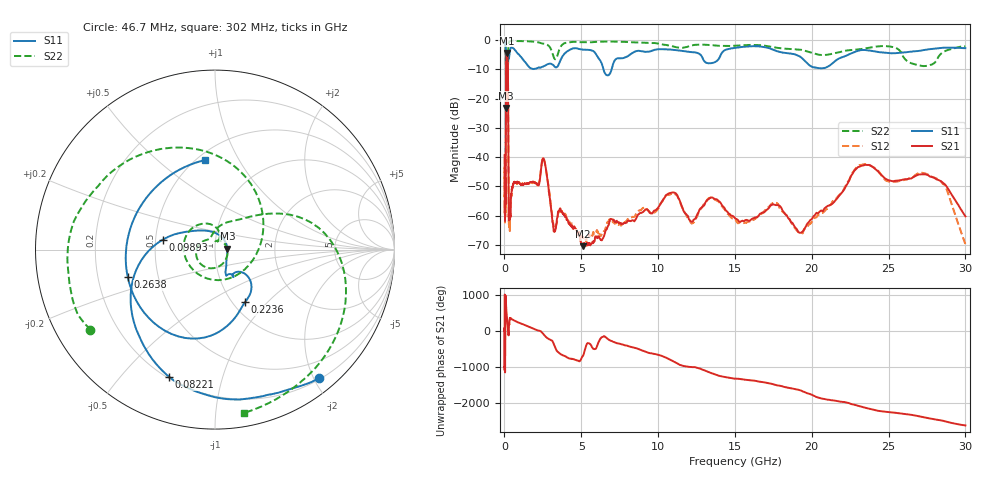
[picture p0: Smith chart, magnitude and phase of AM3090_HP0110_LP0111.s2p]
! Date/Time: Thu, Feb 28, 2019 1:59 PM
! Network Analyzer: Agilent Technologies E8364B Rev: A.07.50.67
! Sweep from 0.010 to 30.000 GHz, 1601 Points, Sweep Type: LOG
! Power Supply: 5.023 V, 0.002 A
# Hz S DB R 50
!freq MagS11 AngS11 MagS21 AngS21 MagS12 AngS12 MagS22 AngS22
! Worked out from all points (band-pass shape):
!   1601 points, 10 MHz to 30 GHz, reference 50 ohm
!   highest |S21| = -4.45 dB at 156 MHz (marker M1); lowest = -70.4 dB at 5.103 GHz (marker M2)
!   |S21| within 3 dB of the highest: 110.9 MHz to 217.7 MHz (106.8 MHz wide, 65 % of centre)
!   lowest |S11| = -23.2 dB at 107.7 MHz (marker M3), VSWR 1.15, Z = 57.4 + j0.698 ohm
!   |S11| at or under -10 dB: 98.52 MHz to 217.9 MHz (119.4 MHz wide, 75.5 % of centre); 6.446 GHz to 6.977 GHz (531.2 MHz wide, 7.91 % of centre)
!   |S22| runs from -28.5 to -0.2 dB; largest |S21 - S12| = 0.015
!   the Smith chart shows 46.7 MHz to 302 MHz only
!   S11 on the Smith chart (normalised r, x): 46.7 MHz: 0.22, -2.08; 82.21 MHz: 0.21, -0.68; 98.93 MHz: 0.55, +0.07; 223.6 MHz: 1.14, -0.75; 263.8 MHz: 0.33, -0.14; 302 MHz: 0.55, +0.73
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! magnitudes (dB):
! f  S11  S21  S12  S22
! 10 MHz  -0.2  -39.3  -49.0  -0.5
! 38.04 MHz  -0.5  -59.8  -61.8  -1.4
! 46.7 MHz  -0.7  -48.1  -51.7  -1.7
! 82.21 MHz  -2.5  -52.0  -53.7  -4.9
! 98.93 MHz  -10.6  -17.5  -17.5  -15.5
! 107.7 MHz  -23.2  -8.7  -8.7  -15.1
! 144.7 MHz  -16.1  -4.6  -4.5  -24.7
! 156 MHz  -15.8  -4.4  -4.4  -22.1
! 223.6 MHz  -9.4  -8.8  -8.8  -13.8
! 263.8 MHz  -5.9  -51.2  -50.2  -1.6
! 302 MHz  -6.0  -60.5  -63.2  -0.7
! 550.5 MHz  -2.8  -49.6  -49.7  -0.3
! 2.084 GHz  -9.8  -48.9  -49.0  -0.7
! 2.558 GHz  -8.9  -40.6  -40.4  -1.3
! 3.22 GHz  -8.8  -65.4  -64.3  -6.1
! 5.103 GHz  -3.3  -70.4  -67.2  -0.8
! 7.926 GHz  -5.9  -62.4  -61.9  -0.7
! 10.86 GHz  -3.3  -52.1  -52.6  -2.1
! 19.41 GHz  -6.4  -65.4  -66.0  -3.5
! 23.59 GHz  -3.5  -42.7  -42.5  -2.8
! 27.83 GHz  -3.1  -46.8  -46.7  -8.4
! 30 GHz  -2.8  -60.2  -69.7  -2.2
